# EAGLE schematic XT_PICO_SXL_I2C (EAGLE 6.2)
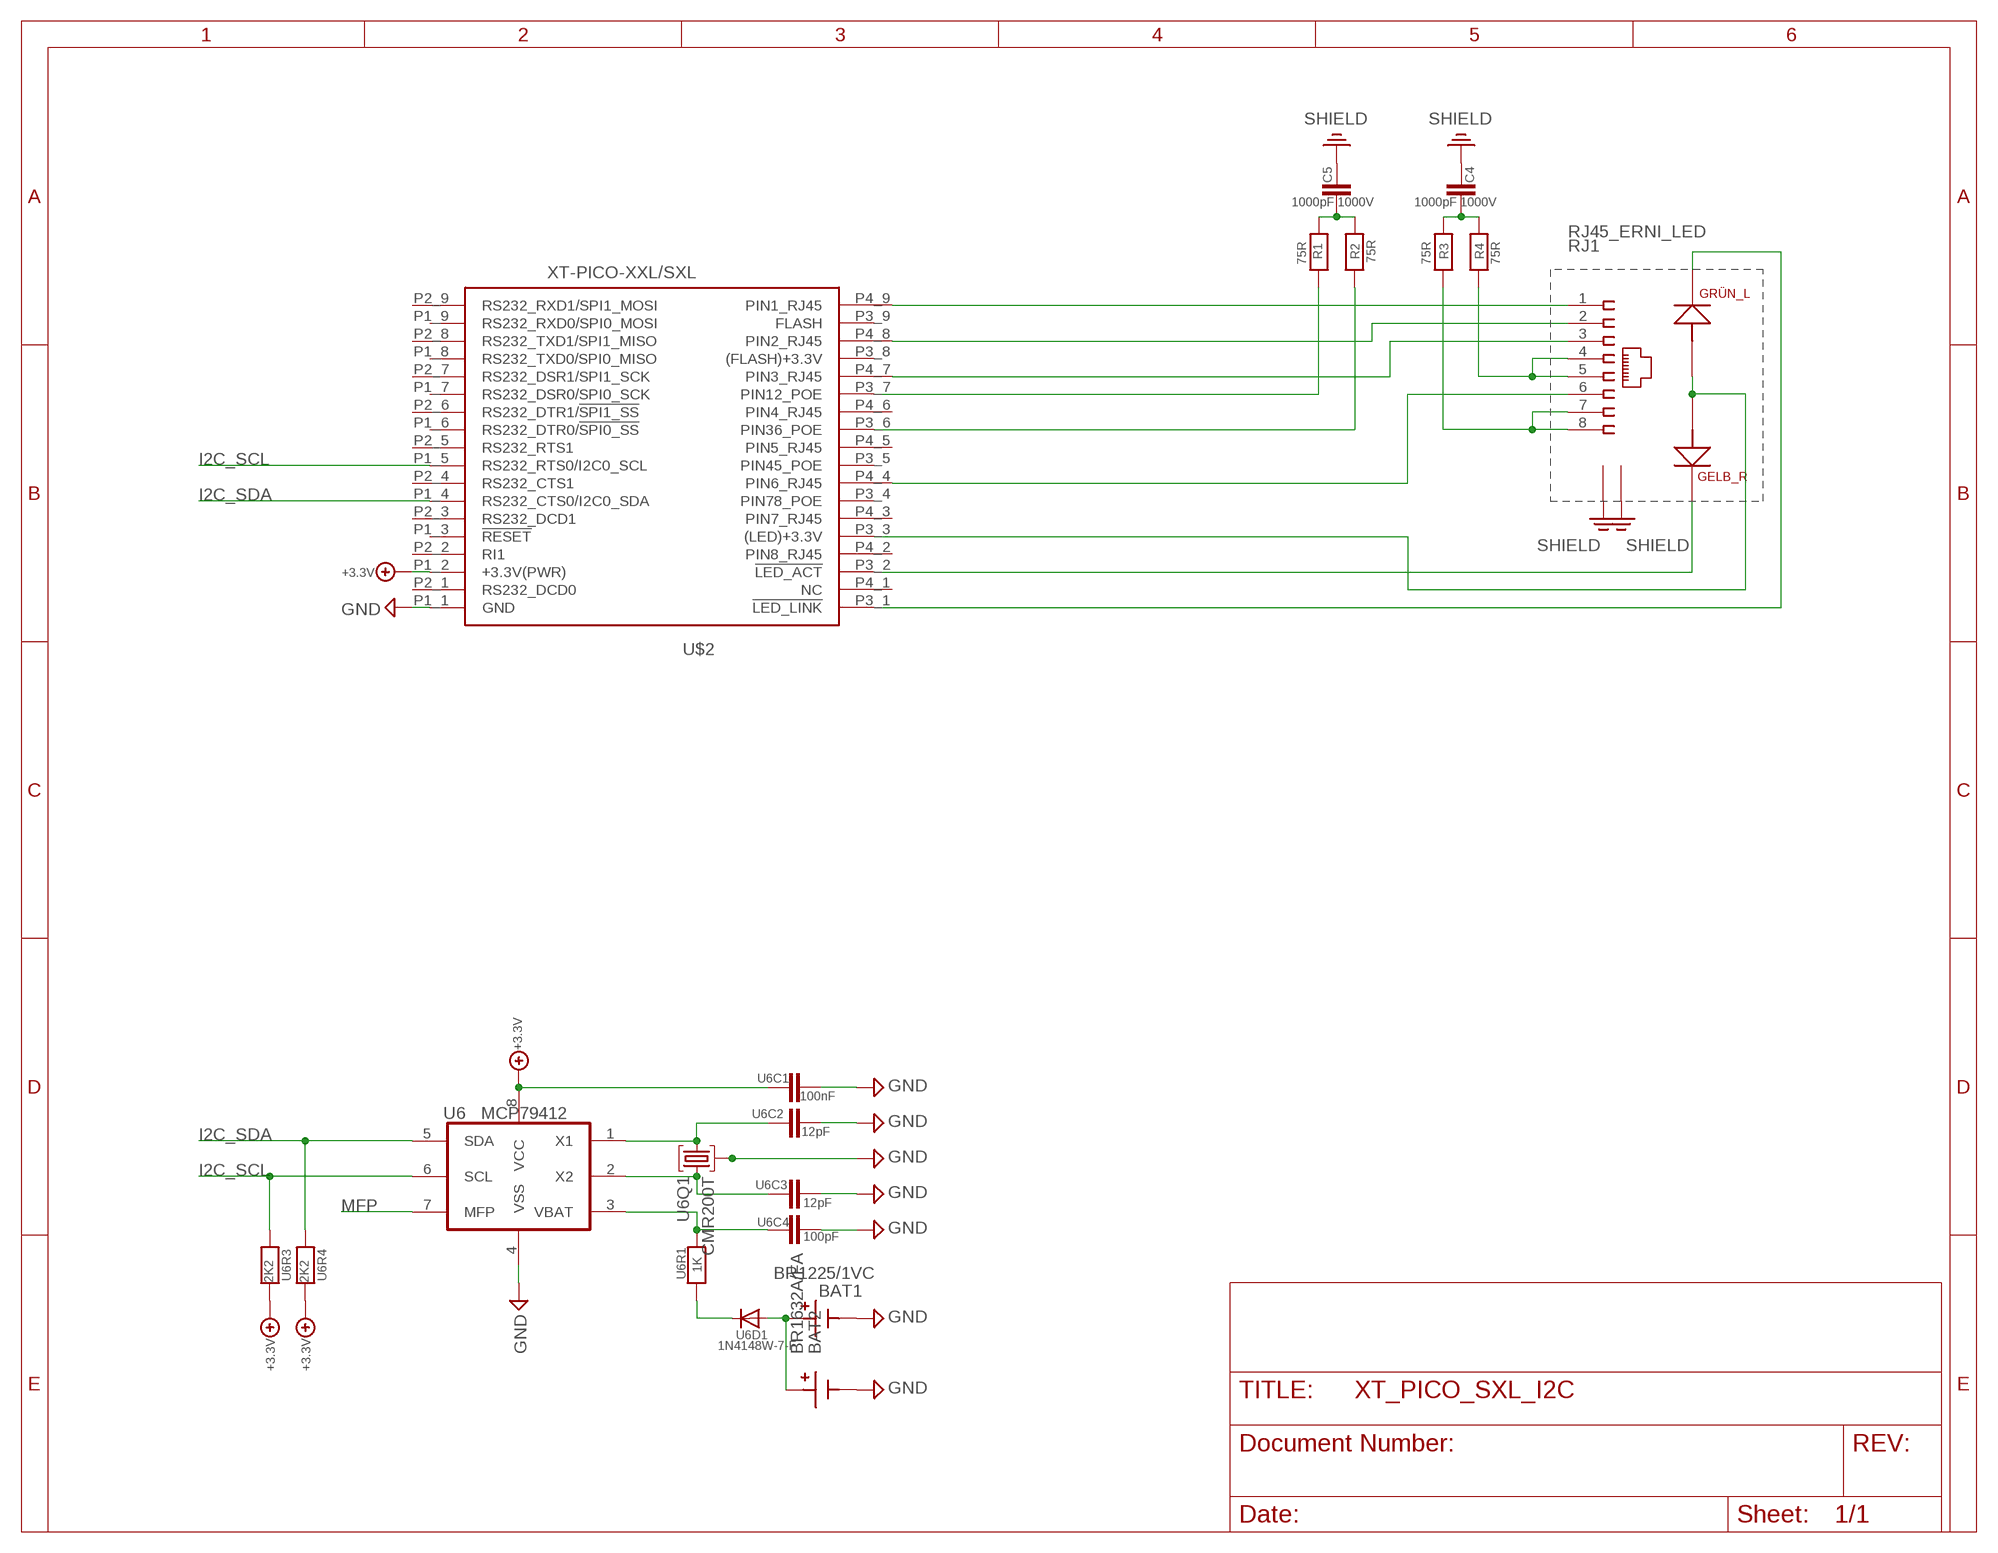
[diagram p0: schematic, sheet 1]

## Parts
BAT1  BR1225/1VC  [BR1225VC]
BAT2  BR1632A/FA  [BR1632A/FA]
C4  1000pF 1000V  CHIP-C-1210  [SMD-1210]
C5  1000pF 1000V  CHIP-C-1210  [SMD-1210]
R1  75R  CHIP-R-0603  [SMD-0603]
R2  75R  CHIP-R-0603  [SMD-0603]
R3  75R  CHIP-R-0603  [SMD-0603]
R4  75R  CHIP-R-0603  [SMD-0603]
RJ1  RJ45_ERNI_LED  [ORCAD_X_ERNI_RJ45_LED]
U6  MCP79412  [SO-8]
U6C1  100nF  CHIP-C-VTS0402  [R0402_VTS]
U6C2  12pF  CHIP-C-VTS0402  [R0402_VTS]
U6C3  12pF  CHIP-C-VTS0402  [R0402_VTS]
U6C4  100pF  CHIP-C-VTS0402  [R0402_VTS]
U6D1  1N4148W-7-F  DIODE-SOD123  [SOD123]
U6Q1  CMR200T  [CMR200T]
U6R1  1K  CHIP-R-VTS04020402_VTS  [R0402_VTS@2]
U6R3  2K2  CHIP-R-VTS04020402_VTS  [R0402_VTS@2]
U6R4  2K2  CHIP-R-VTS04020402_VTS  [R0402_VTS@2]
U$2  XT-PICO-XXL/SXL  [XT-PICO-XXL/SXL]

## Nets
+3.3V: U6.8(VCC) U6C1.1 U6R3.2 U6R4.2 U$2.P1_2(+3.3V(PWR))
GND: BAT1.2 BAT2.P- U6.4(VSS) U6C1.2 U6C2.1 U6C3.1 U6C4.2 U6Q1.EXP U$2.P1_1(GND)
I2C_SCL: U6.6(SCL) U6R3.1 U$2.P1_5(RS232_RTS0/I2C0_SCL)
I2C_SDA: U6.5(SDA) U6R4.1 U$2.P1_4(RS232_CTS0/I2C0_SDA)
MFP: U6.7(MFP)
N$1: R4.2 RJ1.4 RJ1.5
N$2: R3.2 RJ1.7 RJ1.8
N$4: R1.2 U$2.P3_7(PIN12_POE)
N$6: R2.2 U$2.P3_6(PIN36_POE)
N$7: RJ1.1 U$2.P4_9(PIN1_RJ45)
N$8: RJ1.2 U$2.P4_8(PIN2_RJ45)
N$9: RJ1.3 U$2.P4_7(PIN3_RJ45)
N$12: RJ1.6 U$2.P4_4(PIN6_RJ45)
N$15: RJ1.A1 RJ1.A2 U$2.P3_3((LED)+3.3V)
N$16: RJ1.K1 U$2.P3_2(!LED_ACT)
N$17: RJ1.K2 U$2.P3_1(!LED_LINK)
N$19: C4.2 R3.1 R4.1
N$20: C5.1 R1.1 R2.1
N$30: U6.2(X2) U6C3.2 U6Q1.2
N$34: U6.1(X1) U6C2.2 U6Q1.1
N$36: U6.3(VBAT) U6C4.1 U6R1.2
N$45: U6D1.C U6R1.1
N$46: BAT1.1 BAT2.P+ U6D1.A
PE: RJ1.9 RJ1.10 ; supply symbol labelled SHIELD
SHIELD: C4.1 C5.2
Unconnected: U$2.P1_3(!RESET) U$2.P1_6(RS232_DTR0/!SPI0_SS!) U$2.P1_7(RS232_DSR0/SPI0_SCK) U$2.P1_8(RS232_TXD0/SPI0_MISO) U$2.P1_9(RS232_RXD0/SPI0_MOSI) U$2.P2_1(RS232_DCD0) U$2.P2_2(RI1) U$2.P2_3(RS232_DCD1) U$2.P2_4(RS232_CTS1) U$2.P2_5(RS232_RTS1) U$2.P2_6(RS232_DTR1/!SPI1_SS!) U$2.P2_7(RS232_DSR1/SPI1_SCK) U$2.P2_8(RS232_TXD1/SPI1_MISO) U$2.P2_9(RS232_RXD1/SPI1_MOSI) U$2.P3_4(PIN78_POE) U$2.P3_5(PIN45_POE) U$2.P3_8((FLASH)+3.3V) U$2.P3_9(FLASH) U$2.P4_1(NC) U$2.P4_2(PIN8_RJ45) U$2.P4_3(PIN7_RJ45) U$2.P4_5(PIN5_RJ45) U$2.P4_6(PIN4_RJ45)

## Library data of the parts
BAT1 = ak-nord:BR1225/1VC: Panasonic BR-1225/VCN Lithium Battery 3V 48mAh 12,5mm
BAT2 = ak-nord:BR1632A/FA: Panasonic BR1632A/FA Lithium Battery 3V 120mAh d=16mm
C4 C5 = XTMACRO:CHIP-C-?: Chip capacitance
R1-R4 = XTMACRO:CHIP-R-?: Chip resistors
RJ1 = XTMACRO:RJ45_ERNI_LED
U6 = ak-nord:MCP79412: I2C Real-Time Clock/Calendar with EEPROM, SRAM, Unique ID and Battery Switchover
U6C1-U6C4 = mea-lib:CHIP-C-?: Chip capacitance
U6D1 = diode:DIODE-: DIODE
U6Q1 = ak-nord:CMR200T
U6R1 U6R3 U6R4 = mea-lib:CHIP-R-?: Chip resistors
U$2 = ak-devices:XT-PICO-XXL/SXL: AK-NORD XT-PICO-XXL/SXL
